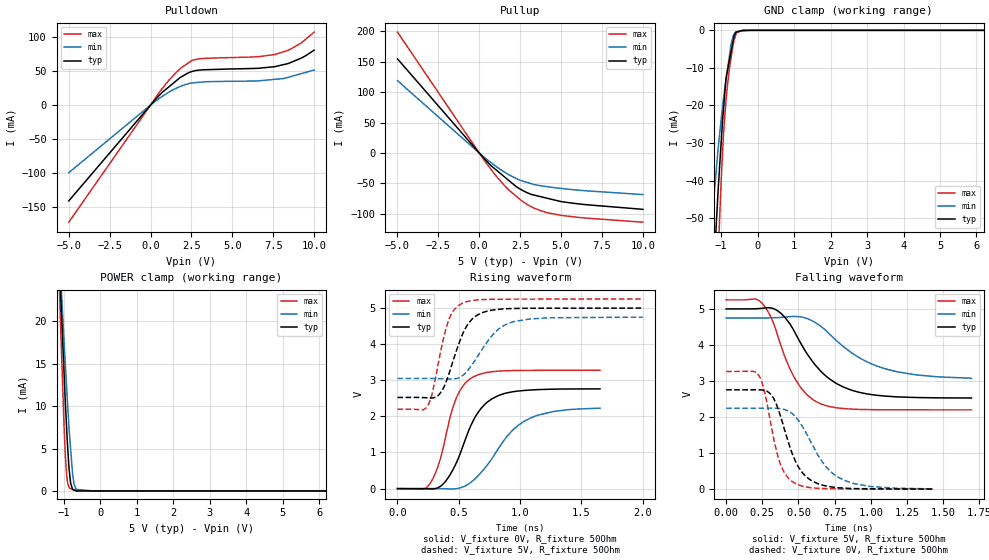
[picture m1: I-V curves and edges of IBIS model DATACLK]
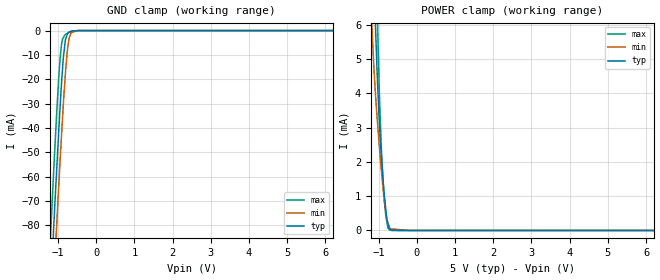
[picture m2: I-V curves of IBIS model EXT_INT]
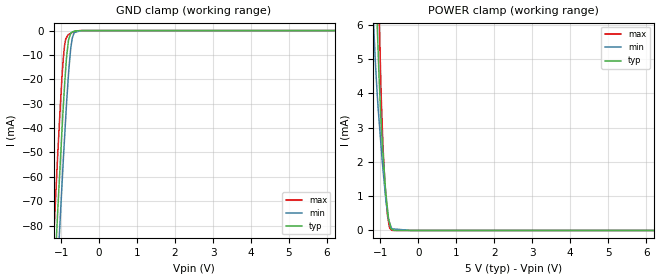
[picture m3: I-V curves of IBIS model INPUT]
|Texas Instruments Incorporated
|12-Bit 40KSPS Analog-to-Digital Converter w/Serial Interface and Reference
|Parallel
| Marketing part#   Digital Voltage Range   Package-type   #pins
| ADS8506IBDW   4.75V to 5.25V   SOIC   28
| ADS8506IBDWG4   4.75V to 5.25V   SOIC   28
| ADS8506IBDWR   4.75V to 5.25V   SOIC   28
| ADS8506IBDWRG4   4.75V to 5.25V   SOIC   28
| ADS8506IDW   4.75V to 5.25V   SOIC   28
| ADS8506IDWG4   4.75V to 5.25V   SOIC   28
| ADS8506IDWR   4.75V to 5.25V   SOIC   28
| ADS8506IDWRG4   4.75V to 5.25V   SOIC   28
[IBIS Ver]   3.2
[File name]   ads8506.ibs
|SIMDE Ver   V2.2 - 201009 - RHL4 - Build 424
[File Rev]   1.1
[Date]   3/16/2011
[Source]
| Texas Instruments Incorporated.
| Analog-eLab Design Center, HPA
| 12500 TI Blvd
| Dallas, TX -75243
| e-mail: elab_ibis@list.ti.com
[Notes]   Revision History:
| Rev 1.0: 3/4/2011
| - Initial version of the model
| - Model generated from simulations in TISPICE
| - Model matched to SPICE simulation
| - C_comp although listed in numerical order of value are
|   obtained from varying PVT conditions. For PVT conditions for
|   each specific value refer the buffer description under
|   respective [Model]. IBIS model user is responsible for using
|   appropriate C_comp to simulate for Signal Integrity.
| - Models are generated with 5V [4.75V and 5.25V].
| - Rleative of ADS8507
| Rev 1.1: 3/16/2011
| - Updated the IBIS model for EXT_INT
[Disclaimer]
| This model is designed as an aid for customers of Texas Instruments.
| TI and its licensors and suppliers make no warranties, either expressed
| or implied, with respect to this  model, including the warranties of
| merchantability or fitness for a particular purpose. The model is
| provided solely on an "as is" basis. The entire risk as to its quality
| and performance is with the customer.
[Copyright]
 (C) Copyright 2011 Texas Instruments Incorporated.All rights reserved.
|   ADS8506
[Component]   ADS8506
[Manufacturer]   TI
[Package]   |28 SOIC  -  DW package
|   typ   min   max
R_pkg   0.18287   0.10984   0.21391
L_pkg   3.80367nH   2.83635nH   6.25153nH
C_pkg   0.71135pF   0.53400pF   1.03462pF
[Pin]  signal_name   model_name   R_pin   L_pin   C_pin
1   R1IN   TERM   0.19580   6.24343nH  1.03405pF
2   AGND1   GND   0.11037   4.50628nH  1.06026pF
3   R2IN   TERM   0.18464   4.13882nH  0.83759pF
4   CAP   TERM   0.10984   3.24437nH  0.71584pF
5   REF   TERM   0.20010   3.40425nH  0.59979pF
6   AGND2   GND   0.09591   2.40375nH  0.61305pF
7   SB/_BTC   INPUT   0.18364   3.17507nH  0.54964pF
8   EXT/_INT   EXT_INT   0.16154   2.83635nH  0.53732pF
9   D7   TRISTATE   0.16460   2.88987nH  0.54628pF
10   D6   TRISTATE   0.18267   3.17264nH  0.58313pF
11   D5   TRISTATE   0.19543   3.38432nH  0.66242pF
12   D4   TRISTATE   0.18546   4.13400nH  0.83694pF
13   D3   TRISTATE   0.18811   5.07798nH  1.02009pF
14   DGND   GND   0.19634   6.26751nH  1.03480pF
15   D2   TRISTATE   0.19459   6.25153nH  1.03462pF
16   D1   TRISTATE   0.18555   5.03697nH  1.01806pF
17   D0   TRISTATE   0.18245   4.06332nH  0.83072pF
18   DATACLK   DATACLK   0.19738   3.49739nH  0.66307pF
19   SDATA   SDATA   0.19964   3.40893nH  0.59620pF
20   TAG   TAG   0.17098   2.99432nH  0.55153pF
21   BYTE   INPUT   0.16046   2.84550nH  0.53400pF
22   R/_C   INPUT   0.16454   2.89455nH  0.53439pF
23   _CS   INPUT   0.18338   3.16884nH  0.55829pF
24   _BUSY   TRISTATE   0.21391   3.63867nH  0.60420pF
25   PWRD   INPUT   0.21327   3.80396nH  0.67779pF
26   REFD   INPUT   0.18801   4.17938nH  0.83520pF
27   VANA   POWER   0.11179   4.53043nH  1.05930pF
28   VDIG   POWER   0.19688   6.28475nH  1.03513pF
29   THERMAL_PAD   NC   0.00002   0.00103nH  3.65811pF
[Model]  TERM
Model_type Terminator
C_comp   1.0e-20F  1.0e-20F  1.0e-20F
|   typ   min   max
[Voltage Range]   5.0V   4.75V   5.25V
[POWER Clamp Reference]   5.0V   4.75V   5.25V
[GND Clamp Reference]   0V   0V   0V
|Ambient Temperature   25   85   -40
|Junction Temperature
[Temperature Range]   25   85   -40
| Models and submodels in the file (7): DATACLK (I/O), EXT_INT (Input), INPUT (Input), SDATA (3-state), TAG (Input), TRISTATE (3-state), TERM (Terminator)
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|   dataclk Model
[Model]   DATACLK
Model_type   I/O
Polarity   Non-Inverting
Enable   Active-Low
Vinl = 0.8
Vinh = 2
Vmeas = 2.5
Vref = 2.5
Cref = 10pF
Rref = 50
|   typ   min   max
|   (nom PVT)   (Fast PVT)   (slow PVT)
|C_comp from frequency method(29MHz)
|Average
C_comp   3.527e-12   2.938e-12   4.119e-12
|ON state : BUFFER OUTPUT TURNED HIGH
|C_comp   3.711e-12   3.139e-12   4.318e-12
|OFF state: BUFFER IN HIGH IMPEDANCE
|C_comp   3.343e-12   2.737e-12   3.920e-12
|C_comp from LC tank measurement(L=1nH)
|Average
|Resonant Frequency(Hz)   3.000e+09   3.185e+09   2.890e+09
|C_comp   2.824e-12   2.509e-12   3.039e-12
|ON state : BUFFER OUTPUT TURNED HIGH
|Resonant Frequency(Hz)   2.920e+09   3.070e+09   2.840e+09
|C_comp   2.974e-12   2.690e-12   3.144e-12
|OFF state: BUFFER IN HIGH IMPEDANCE
|Resonant Frequency(Hz)   3.080e+09   3.300e+09   2.940e+09
|C_comp   2.673e-12   2.328e-12   2.933e-12
| Where nom  PVT is Nominal Process,  5V,  25C
|   Fast PVT is Strong Process,   5.25V,  -40C
|   Slow PVT is Weak Process,   4.75V,  85C
[Voltage Range]   5   4.75   5.25
|Ambient Temperature   25   85   -40
|Junction Temperature
[Temperature Range]   25   85   -40
[Pullup Reference]   5   4.75   5.25
[Pulldown Reference]   0   0   0
[Power Clamp Reference]   5   4.75   5.25
[GND Clamp Reference]   0   0   0
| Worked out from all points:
|   slope of the pulldown table from 0 to 0.75 V, typ, clamps not added: 38.6 ohm
|   slope of the pullup table from 0 to 0.75 V, typ, clamps not added: 34.9 ohm
|   GND clamp passes 1 mA (typ) near -0.62 V on its own axis
|   POWER clamp passes 1 mA (typ) near -0.82 V on its own axis
|   falling waveform, V_fixture 5V, R_fixture 50Ohm: 20-80 % time 275ps typ, 360ps min, 194ps max; typ from 5 V to 2.53 V
|   rising waveform, V_fixture 0V, R_fixture 50Ohm: 20-80 % time 222ps typ, 315ps min, 161ps max; typ from 0 V to 2.76 V
|   rising waveform, V_fixture 5V, R_fixture 50Ohm: 20-80 % time 162ps typ, 222ps min, 120ps max; typ from 2.52 V to 5 V
|   falling waveform, V_fixture 0V, R_fixture 50Ohm: 20-80 % time 149ps typ, 213ps min, 109ps max; typ from 2.76 V to 0.006 V
[Pulldown]
|   Voltage   I(typ)   I(min)   I(max)
-5V       -141.2mA   -99.65mA   -172.6mA
255mV     7.087mA    4.92mA     8.994mA
700mV     18.42mA    12.51mA    23.9mA
1.145V    27.31mA    19.44mA    37.2mA
1.906V    41.92mA    28.28mA    55.49mA
2.551V    49.63mA    32.64mA    66mA
2.94V     51.44mA    33.43mA    68.06mA
6.557V    54.15mA    35.59mA    71.22mA
7.591V    56.54mA    37.88mA    74.4mA
8.442V    61.44mA    41.08mA    80.94mA
9.229V    69.37mA    46.44mA    91.74mA
10V       80.82mA    51.68mA    107.5mA
[GND Clamp]
|   Voltage   I(typ)   I(min)   I(max)
-5V       -886.3mA   -642.9mA   -1.225A
-1.306V   -82.7mA    -56.49mA   -121.5mA
-1.176V   -59.29mA   -41.92mA   -84.92mA
-1.071V   -40.73mA   -30.46mA   -57.11mA
-997.5mV  -29.5mA    -23.49mA   -39.66mA
-934.5mV  -20.79mA   -18.27mA   -27.63mA
-866.2mV  -12.81mA   -13.14mA   -18.44mA
-726.8mV  -5.65mA    -3.64mA    -7.319mA
-640mV    -1.252mA   -988.4uA   -2.453mA
-598.5mV  -634.3uA   -346uA     -1.157mA
-393.7mV  -5.447uA   -172.6uA   -2.515uA
10V       0A         0A         0A
[Pullup]
|   Voltage   I(typ)   I(min)   I(max)
-5V       154.7mA    118.9mA    198.7mA
409.5mV   -12.21mA   -9.375mA   -15.99mA
1.076V    -28.81mA   -23.13mA   -39.34mA
1.596V    -40.46mA   -32.36mA   -55.04mA
2.27V     -55.56mA   -42.15mA   -71.34mA
2.63V     -61.26mA   -46.07mA   -79.42mA
3.165V    -68.02mA   -50.33mA   -88.09mA
3.838V    -72.38mA   -54.2mA    -95.66mA
4.956V    -79.64mA   -58.13mA   -102.3mA
6.565V    -85.13mA   -62.24mA   -107.1mA
10V       -92.7mA    -68.39mA   -113.8mA
[POWER Clamp]
|   Voltage   I(typ)   I(min)   I(max)
-5V       172mA      157.5mA    190.5mA
-1.306V   46.79mA    43.79mA    49.91mA
-1.092V   23.83mA    25.73mA    19.93mA
-1.085V   23.07mA    25.14mA    19.05mA
-1.016V   16.24mA    19.51mA    10.51mA
-987mV    13.31mA    17.16mA    6.931mA
-918.7mV  7.036mA    11.91mA    1.708mA
-865mV    3.122mA    7.948mA    558.9uA
-815mV    973.1uA    5.044mA    273.2uA
-755.2mV  173.5uA    1.847mA    180uA
-665mV    9.017uA    183uA      39.33uA
10V       0A         0A         0A
[Ramp]
R_load = 50
|   typ   min   max
dV/dt_r   1.65757/2.22157e-10   1.34454/3.17426e-10   1.96633/1.60464e-10
dV/dt_f   1.48329/2.74262e-10   1.01323/3.67973e-10   1.83011/1.93734e-10
[Falling Waveform]
V_fixture = 5V
V_fixture_min = 4.75V
V_fixture_max = 5.25V
R_fixture = 50Ohm
|   Time   V(typ)   V(min)   V(max)
0s        5V         4.75V      5.25V
248.5ps   5.016V     4.749V     5.157V
306.2ps   5.027V     4.751V     4.8V
363.3ps   4.926V     4.76V      4.167V
475.4ps   4.346V     4.79V      3.07V
556.5ps   3.775V     4.737V     2.631V
645.9ps   3.307V     4.544V     2.382V
809.2ps   2.836V     3.959V     2.238V
1.042ns   2.605V     3.417V     2.205V
1.696ns   2.53V      3.078V     2.2V
[Rising Waveform]
V_fixture = 0V
V_fixture_min = 0V
V_fixture_max = 0V
R_fixture = 50Ohm
|   Time   V(typ)   V(min)   V(max)
0s        1.852nV    2.174nV    1.648nV
265.3ps   -8.871mV   675.1uV    135.4mV
349.1ps   61.16mV    -1.796mV   818mV
478.4ps   701mV      -1.803mV   2.498V
615.2ps   1.867V     220.1mV    3.089V
772.1ps   2.49V      840.3mV    3.238V
902.4ps   2.659V     1.485V     3.266V
1.033ns   2.718V     1.865V     3.273V
1.269ns   2.754V     2.134V     3.276V
1.651ns   2.762V     2.229V     3.277V
[Rising Waveform]
V_fixture = 5V
V_fixture_min = 4.75V
V_fixture_max = 5.25V
R_fixture = 50Ohm
|   Time   V(typ)   V(min)   V(max)
0s        2.524V     3.051V     2.198V
244.7ps   2.514V     3.052V     2.282V
282.3ps   2.508V     3.05V      2.626V
335.9ps   2.59V      3.046V     3.522V
410.2ps   3.086V     3.034V     4.595V
531.4ps   4.283V     3.132V     5.137V
646.2ps   4.798V     3.626V     5.224V
787.4ps   4.951V     4.301V     5.244V
912.2ps   4.985V     4.585V     5.247V
2ns       4.999V     4.748V     5.249V
[Falling Waveform]
V_fixture = 0V
V_fixture_min = 0V
V_fixture_max = 0V
R_fixture = 50Ohm
|   Time   V(typ)   V(min)   V(max)
0s        2.756V     2.246V     3.265V
228.2ps   2.756V     2.247V     3.142V
266.4ps   2.737V     2.249V     2.69V
306.4ps   2.64V      2.249V     1.876V
373.1ps   2.063V     2.234V     720.3mV
476.7ps   798.9mV    2.023V     164.1mV
581.2ps   263mV      1.345V     45.67mV
688.4ps   93.17mV    633.4mV    18.13mV
774.9ps   43.22mV    333.5mV    11.53mV
1.43ns    6.228mV    11.01mV    2.715mV
|   ext_int Model
[Model]   EXT_INT
Model_type   Input
Vinl = 0.8
Vinh = 2
|   typ   min   max
|   (nom PVT)   (Fast PVT)   (slow PVT)
|C_comp from frequency method(29MHz)
|Average
|C_comp   1.100e-12   9.944e-13   1.209e-12
|C_comp from LC tank measurement(L=1nH)
|Resonant Frequency(Hz)   5.450e+09   5.580e+09   5.360e+09
C_comp   8.536e-13   8.143e-13   8.826e-13
| Where nom  PVT is Nominal Process,  5V,  25C
|   Fast PVT is Strong Process,   5.25V,  -40C
|   Slow PVT is Weak Process,   4.75V,  85C
[Voltage Range]   5   4.75   5.25
|Ambient Temperature   25   85   -40
|Junction Temperature
[Temperature Range]   25   85   -40
[Power Clamp Reference]   5   4.75   5.25
[GND Clamp Reference]   0   0   0
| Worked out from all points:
|   GND clamp passes 1 mA (typ) near -0.74 V on its own axis
|   POWER clamp passes 1 mA (typ) near -0.85 V on its own axis
[GND Clamp]
|   Voltage   I(typ)   I(min)   I(max)
-5V       -1.41A     -1.422A    -1.398A
-1.306V   -143.6mA   -166.2mA   -120.7mA
-1.103V   -78.34mA   -101.3mA   -54.93mA
-1.08V    -71.2mA    -94.3mA    -48.17mA
-1.036V   -58.09mA   -80.63mA   -34.93mA
-939.7mV  -30.38mA   -52.33mA   -10.86mA
-903mV    -20.97mA   -42.31mA   -5.391mA
-855mV    -10.66mA   -29.38mA   -2.776mA
-805mV    -3.827mA   -17.8mA    -1.643mA
-745.8mV  -1.139mA   -7.141mA   -1.117mA
-640mV    -142.4uA   -741.4uA   -244.7uA
10V       0A         0A         0A
[POWER Clamp]
|   Voltage   I(typ)   I(min)   I(max)
-5V       203.6mA    171.5mA    247.6mA
-1.178V   10.1mA     6.068mA    14mA
-1.075V   5.805mA    3.891mA    8.406mA
-1.035V   4.546mA    3.266mA    6.432mA
-990mV    3.395mA    2.616mA    4.489mA
-971.2mV  3.013mA    2.345mA    3.744mA
-929.3mV  2.25mA     1.79mA     2.441mA
-876.8mV  1.416mA    1.165mA    1.332mA
-813.7mV  656.9uA    564.7uA    459.3uA
-756mV    219.4uA    225.4uA    72.66uA
-698.3mV  41.75uA    49.25uA    5.693uA
10V       0A         0A         0A
|   input Model
[Model]   INPUT
Model_type   Input
Vinl = 0.8
Vinh = 2
|   typ   min   max
|   (nom PVT)   (Fast PVT)   (slow PVT)
|C_comp from frequency method(29MHz)
|Average
|C_comp   1.101e-12   9.946e-13   1.209e-12
|C_comp from LC tank measurement(L=1nH)
|Resonant Frequency(Hz)   5.460e+09   5.580e+09   5.370e+09
C_comp   8.505e-13   8.143e-13   8.793e-13
| Where nom  PVT is Nominal Process,  5V,  25C
|   Fast PVT is Strong Process,   5.25V,  -40C
|   Slow PVT is Weak Process,   4.75V,  85C
[Voltage Range]   5   4.75   5.25
|Ambient Temperature   25   85   -40
|Junction Temperature
[Temperature Range]   25   85   -40
[Power Clamp Reference]   5   4.75   5.25
[GND Clamp Reference]   0   0   0
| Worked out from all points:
|   GND clamp passes 1 mA (typ) near -0.74 V on its own axis
|   POWER clamp passes 1 mA (typ) near -0.85 V on its own axis
[GND Clamp]
|   Voltage   I(typ)   I(min)   I(max)
-5V       -1.41A     -1.421A    -1.398A
-1.306V   -143.5mA   -166.1mA   -120.6mA
-1.103V   -78.32mA   -101.3mA   -54.9mA
-1.08V    -71.17mA   -94.27mA   -48.15mA
-1.036V   -58.07mA   -80.61mA   -34.91mA
-939.7mV  -30.37mA   -52.31mA   -10.85mA
-903mV    -20.96mA   -42.29mA   -5.382mA
-855mV    -10.66mA   -29.37mA   -2.769mA
-805mV    -3.822mA   -17.8mA    -1.638mA
-745.8mV  -1.137mA   -7.136mA   -1.114mA
-640mV    -142.1uA   -740.2uA   -244uA
10V       0A         0A         0A
[POWER Clamp]
|   Voltage   I(typ)   I(min)   I(max)
-5V       203.3mA    171.3mA    247.3mA
-1.178V   10.07mA    6.04mA     13.97mA
-1.075V   5.787mA    3.871mA    8.393mA
-1.035V   4.532mA    3.248mA    6.423mA
-990mV    3.384mA    2.601mA    4.484mA
-971.2mV  3.004mA    2.332mA    3.74mA
-929.3mV  2.244mA    1.78mA     2.44mA
-876.8mV  1.413mA    1.158mA    1.332mA
-813.7mV  656uA      560.8uA    459.3uA
-756mV    219.3uA    223.8uA    72.66uA
-698.3mV  41.74uA    49.02uA    5.692uA
10V       0A         0A         0A
